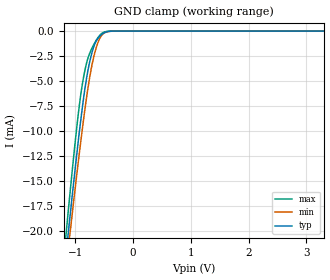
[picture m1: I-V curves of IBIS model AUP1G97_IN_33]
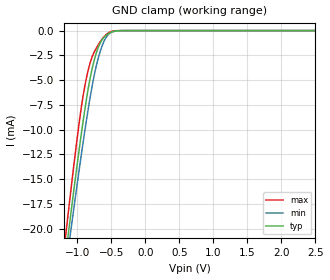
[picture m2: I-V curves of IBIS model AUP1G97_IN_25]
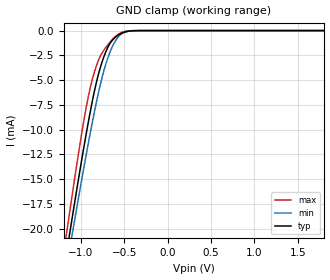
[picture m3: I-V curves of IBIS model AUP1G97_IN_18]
| TEXAS INSTRUMENTS INCORPORATED
| Standard Linear and Logic Group
| IBIS Model of SN74AUP1G97
| Low-power Configurable Multiple-Function Gate
| This file contains package information for the following:
|  SOT 6-pin (DBV) package as [Component] AUP1G97_DBV
|  SOT 6-pin (DCK) package as [Component] AUP1G97_DCK
|  DSBGA 6-pin (YEP_YZP) package as [Component] AUP1G97_YEP_YZP
| This device can be powered at the following Vccs:
|  3.3 volt Vcc
|  2.5 volt Vcc
|  1.8 volt Vcc
|  1.5 volt Vcc
|  1.2 volt Vcc
|  0.8 volt Vcc
| This file provides unique models under the [Model Selector] for each Vcc.
| For operation at a specific Vcc, select the appropriate model after each
| [Model Selector] keyword.
[IBIS Ver]   3.2
[Comment char]  |_char
[File Name]   sn74aup1g97.ibs
[File Rev]   1.2 | a_die
[Date]   August 26, 2004
[Source]   Data created from TI-SPICE simulations at TI-SLL.
[Notes]   The following is an IBIS list for the AUP1G97.
   Please contact sllibis@ti.com with questions and
   comments concerning SLL IBIS models.
   - FILE REV HISTORY
   - 1.1 Release IBIS file on 12/3/2003
   - 1.2 YEP and YZP packages released on 08/26/04
   - Power clamp data deleted as there is no power-clamp diode.
   - Non-monotonic data in pullup data due to resistor at output.
[Disclaimer] Property of Texas Instruments Incorporated.  Unauthorized
   reproduction and/or distribution is strictly prohibited.
   This product is protected under copyright law.
   Created  2003, (C) Copyright  2003, Texas Instruments
   Incorporated, All Rights Reserved
   UNLESS THERE IS A SIGNED, WRITTEN AGREEMENT TO THE
   CONTRARY, TEXAS INSTRUMENTS (TI) IS PROVIDING THE IBIS
   MODELS  AND WITHOUT ANY WARRANTY, EXPRESSED OR
   IMPLIED.  TI assumes no liability for:
   1) the accuracy of the IBIS models provided to your
   company;
   2) the proper functioning of these IBIS Models in your
   design or for any resulting applications; or
   3) infringement of patents, copyrights or intellectual
   property rights resulting from your use of these IBIS
   models.
   TI provides IBIS Models as a service to our customers.
   You and your company shall not distribute, sell or give
   these models to anyone else without prior written
   permission from TI.
   TI reserves the right to make changes to our products or
   to discontinue any semiconductor product or service
   without notice, and advises our customers to obtain the
   latest version of relevant information to verify, before
   placing orders, that the information being relied on is
   current.
   Please be aware that your receipt and use of the IBIS
   information provided shall serve as acceptance of these
   terms and conditions.  If you do not accept these terms,
   you should return or destroy the IBIS models and any
   other accompanying information immediately.
| Component AUP1G97_DBV 6-pin SOT
[Component]   AUP1G97_DBV
[Manufacturer]   Texas Instruments, Inc.
[Package]
|   typ   min   max
R_pkg   2.500e-02   1.900e-02   3.700e-02
L_pkg   1.524e-09   1.260e-09   1.751e-09
C_pkg   2.450e-13   1.980e-13   2.640e-13
[Pin]   signal_name   model_name   R_pin   L_pin   C_pin
1   B   AUP1G97_IN   2.100e-02   1.405e-09   2.460e-13
2   GND   GND   3.700e-02   1.751e-09   2.630e-13
3   A   AUP1G97_IN   2.600e-02   1.493e-09   2.470e-13
4   Y   AUP1G97_OUT   1.900e-02   1.620e-09   2.640e-13
5   VCC   POWER   2.400e-02   1.260e-09   1.980e-13
6   C   AUP1G97_IN   2.100e-02   1.617e-09   2.500e-13
| Component AUP1G97_DCK 6-pin SOT
[Component]   AUP1G97_DCK
[Manufacturer]   Texas Instruments, Inc.
[Package]
|   typ   min   max
R_pkg   1.400e-02   1.100e-02   2.100e-02
L_pkg   9.480e-10   7.840e-10   1.103e-09
C_pkg   1.910e-13   1.670e-13   2.050e-13
[Pin]   signal_name   model_name   R_pin   L_pin   C_pin
1   B   AUP1G97_IN   1.300e-02   9.840e-10   1.960e-13
2   GND   GND   2.100e-02   1.103e-09   2.050e-13
3   A   AUP1G97_IN   1.100e-02   9.980e-10   1.970e-13
4   Y   AUP1G97_OUT   1.300e-02   9.040e-10   1.900e-13
5   VCC   POWER   1.500e-02   7.840e-10   1.670e-13
6   C   AUP1G97_IN   1.200e-02   9.160e-10   1.950e-13
| Component AUP1G97_YEP_YZP 6-pin DSBGA
[Component]   AUP1G97_YEP_YZP
[Manufacturer]   Texas Instruments, Inc.
[Package]
|   typ   min   max
R_pkg   1.000e-03   1.000e-03   2.100e-02
L_pkg   2.450e-11   2.400e-11   1.103e-09
C_pkg   5.600e-14   0.000e+00   2.050e-13
[Pin]   signal_name   model_name   R_pin   L_pin   C_pin
1   B   AUP1G97_IN   1.000e-03   2.500e-11   6.400e-14
2   GND   GND   1.000e-03   2.400e-11   6.700e-14
3   A   AUP1G97_IN   1.000e-03   2.500e-11   6.400e-14
4   Y   AUP1G97_OUT   1.000e-03   2.500e-11   6.400e-14
5   VCC   POWER   1.000e-03   2.400e-11   6.700e-14
6   C   AUP1G97_IN   1.000e-03   2.500e-11   6.400e-14
| Model AUP1G97_IN
[Model Selector]   AUP1G97_IN
AUP1G97_IN_33   3.3 volt Vcc
AUP1G97_IN_25   2.5 volt Vcc
AUP1G97_IN_18   1.8 volt Vcc
AUP1G97_IN_15   1.5 volt Vcc
AUP1G97_IN_12   1.2 volt Vcc
AUP1G97_IN_08   0.8 volt Vcc
| Model AUP1G97_OUT
[Model Selector]   AUP1G97_OUT
AUP1G97_OUT_33   3.3 volt Vcc
AUP1G97_OUT_25   2.5 volt Vcc
AUP1G97_OUT_18   1.8 volt Vcc
AUP1G97_OUT_15   1.5 volt Vcc
AUP1G97_OUT_12   1.2 volt Vcc
AUP1G97_OUT_08   0.8 volt Vcc
| Models and submodels in the file (12): AUP1G97_IN_33 (Input), AUP1G97_IN_25 (Input), AUP1G97_IN_18 (Input), AUP1G97_IN_15 (Input), AUP1G97_IN_12 (Input), AUP1G97_IN_08 (Input), AUP1G97_OUT_33 (Output), AUP1G97_OUT_25 (Output), AUP1G97_OUT_18 (Output), AUP1G97_OUT_15 (Output), AUP1G97_OUT_12 (Output), AUP1G97_OUT_08 (Output)
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[Model]   AUP1G97_IN_33
Model_type  Input
Vinl=0.9
Vinh=2
| variable   typ   min   max
C_comp   1.43pF   1.18pF   1.80pF
[Temperature Range]   40   100   -40
| Ambient temperature   25   85   -40
[Voltage range]   3.3   3   3.6
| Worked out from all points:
|   GND clamp passes 1 mA (typ) near -0.64 V on its own axis
[GND Clamp]
| AUP1G97_IN_33
|   Voltage   I(typ)   I(min)   I(max)
-3.6V     -171.6mA   -163.5mA   -181.1mA
-1.16V    -22.22mA   -23.69mA   -20.18mA
-1.11V    -19.45mA   -21.09mA   -17.19mA
-1.085V   -18.08mA   -19.81mA   -15.71mA
-940mV    -10.5mA    -12.6mA    -7.822mA
-890mV    -8.117mA   -10.26mA   -5.698mA
-835mV    -5.768mA   -7.825mA   -3.925mA
-755mV    -3.153mA   -4.717mA   -2.255mA
-675mV    -1.463mA   -2.419mA   -1.277mA
-595mV    -617.7uA   -945.8uA   -546.7uA
-515mV    -215.4uA   -248.8uA   -134.4uA
3.3V      132.2pA    540.4pA    36.28pA
[Model]   AUP1G97_IN_25
Model_type  Input
Vinl=0.7
Vinh=1.6
| variable   typ   min   max
C_comp   1.47pF   1.22pF   1.79pF
[Temperature Range]   40   100   -40
| Ambient temperature   25   85   -40
[Voltage range]   2.5   2.3   2.7
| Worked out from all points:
|   GND clamp passes 1 mA (typ) near -0.64 V on its own axis
[GND Clamp]
| AUP1G97_IN_25
|   Voltage   I(typ)   I(min)   I(max)
-3.6V     -171.6mA   -163.5mA   -181.1mA
-1.165V   -22.5mA    -23.95mA   -20.48mA
-1.115V   -19.72mA   -21.35mA   -17.49mA
-1.09V    -18.36mA   -20.06mA   -16.01mA
-945mV    -10.75mA   -12.84mA   -8.061mA
-890mV    -8.117mA   -10.26mA   -5.698mA
-835mV    -5.768mA   -7.825mA   -3.925mA
-760mV    -3.287mA   -4.89mA    -2.329mA
-675mV    -1.463mA   -2.419mA   -1.277mA
-595mV    -617.7uA   -945.8uA   -546.7uA
-520mV    -233.1uA   -272.6uA   -149.9uA
2.5V      104.3pA    491.9pA    26.71pA
[Model]   AUP1G97_IN_18
Model_type  Input
Vinl=0.6825
Vinh=1.0725
| variable   typ   min   max
C_comp   1.51pF   1.28pF   1.78pF
[Temperature Range]   40   100   -40
| Ambient temperature   25   85   -40
[Voltage range]   1.8   1.65   1.95
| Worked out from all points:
|   GND clamp passes 1 mA (typ) near -0.64 V on its own axis
[GND Clamp]
| AUP1G97_IN_18
|   Voltage   I(typ)   I(min)   I(max)
-3.6V     -171.6mA   -163.5mA   -181.1mA
-1.16V    -22.22mA   -23.69mA   -20.18mA
-1.135V   -20.83mA   -22.39mA   -18.68mA
-1.11V    -19.45mA   -21.09mA   -17.19mA
-1.09V    -18.36mA   -20.06mA   -16.01mA
-960mV    -11.5mA    -13.57mA   -8.799mA
-850mV    -6.372mA   -8.471mA   -4.359mA
-780mV    -3.86mA    -5.615mA   -2.659mA
-710mV    -2.096mA   -3.313mA   -1.67mA
-625mV    -855.5uA   -1.409mA   -788.9uA
-540mV    -313.2uA   -390uA     -224.9uA
1.8V      83.14pA    451.3pA    18.98pA
